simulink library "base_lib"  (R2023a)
settings: Solver=VariableStepAuto  StartTime=0.0  StopTime=10.0  RelTol=1e-3
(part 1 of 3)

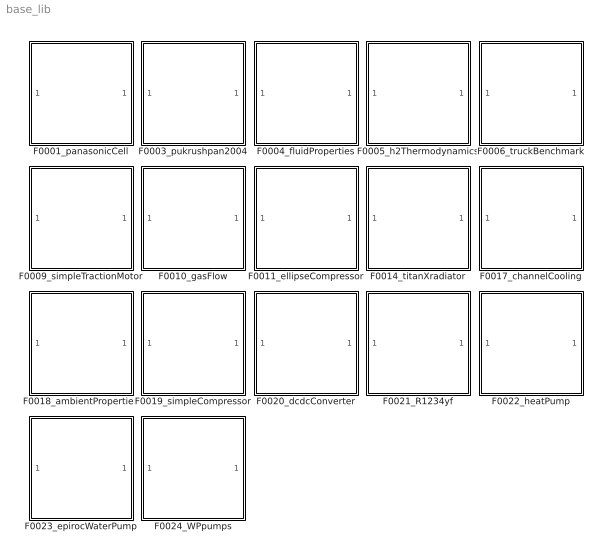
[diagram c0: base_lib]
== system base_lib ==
  F0001_panasonicCell : Subsystem
  F0003_pukrushpan2004 : Subsystem
  F0004_fluidProperties : Subsystem
  F0005_h2Thermodynamics : Subsystem
  F0006_truckBenchmark : Subsystem
  F0009_simpleTractionMotor : Subsystem
  F0010_gasFlow : Subsystem
  F0011_ellipseCompressor : Subsystem
  F0014_titanXradiator : Subsystem
  F0017_channelCooling : Subsystem
  F0018_ambientProperties : Subsystem
  F0019_simpleCompressor : Subsystem
  F0020_dcdcConverter : Subsystem
  F0021_R1234yf : Subsystem
  F0022_heatPump : Subsystem
  F0023_epirocWaterPump : Subsystem
  F0024_WPpumps : Subsystem

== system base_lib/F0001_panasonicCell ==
  F0001_cellCapacity.m : MATLAB Function  TreatAsAtomicUnit=on
  F0001_dynamicVoltage.m : MATLAB Function  TreatAsAtomicUnit=on
  F0001_ocvSOC.m : MATLAB Function  TreatAsAtomicUnit=on

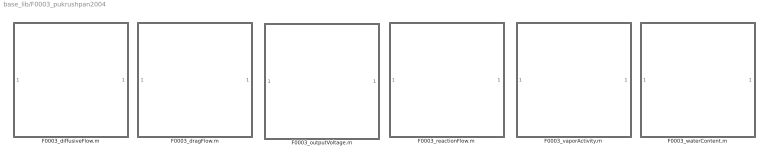
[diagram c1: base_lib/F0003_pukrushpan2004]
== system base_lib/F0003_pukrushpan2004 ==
  F0003_diffusiveFlow.m : MATLAB Function  TreatAsAtomicUnit=on
  F0003_dragFlow.m : MATLAB Function  TreatAsAtomicUnit=on
  F0003_outputVoltage.m : MATLAB Function  TreatAsAtomicUnit=on
  F0003_reactionFlow.m : MATLAB Function  TreatAsAtomicUnit=on
  F0003_vaporActivity.m : MATLAB Function  TreatAsAtomicUnit=on
  F0003_waterContent.m : MATLAB Function  TreatAsAtomicUnit=on

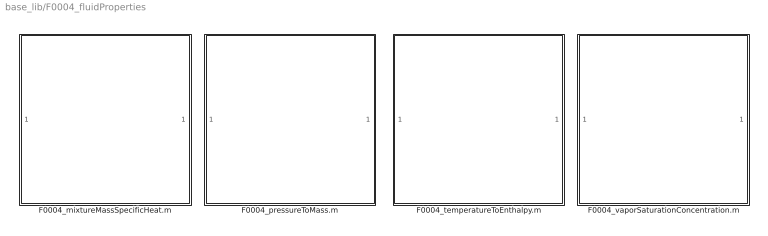
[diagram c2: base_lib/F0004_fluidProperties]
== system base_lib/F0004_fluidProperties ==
  F0004_mixtureMassSpecificHeat.m : MATLAB Function  TreatAsAtomicUnit=on
  F0004_pressureToMass.m : MATLAB Function  TreatAsAtomicUnit=on
  F0004_temperatureToEnthalpy.m : MATLAB Function  TreatAsAtomicUnit=on
  F0004_vaporSaturationConcentration.m : MATLAB Function  TreatAsAtomicUnit=on

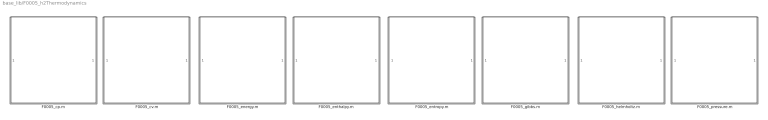
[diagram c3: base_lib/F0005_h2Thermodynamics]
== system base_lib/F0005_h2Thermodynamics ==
  F0005_cp.m : MATLAB Function  TreatAsAtomicUnit=on
  F0005_cv.m : MATLAB Function  TreatAsAtomicUnit=on
  F0005_energy.m : MATLAB Function  TreatAsAtomicUnit=on
  F0005_enthalpy.m : MATLAB Function  TreatAsAtomicUnit=on
  F0005_entropy.m : MATLAB Function  TreatAsAtomicUnit=on
  F0005_gibbs.m : MATLAB Function  TreatAsAtomicUnit=on
  F0005_helmholtz.m : MATLAB Function  TreatAsAtomicUnit=on
  F0005_pressure.m : MATLAB Function  TreatAsAtomicUnit=on

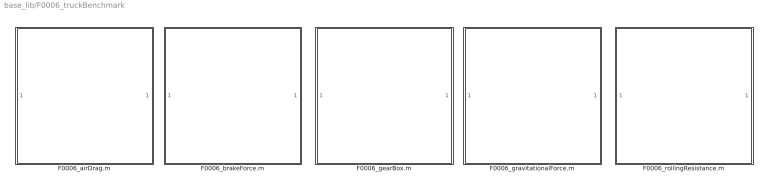
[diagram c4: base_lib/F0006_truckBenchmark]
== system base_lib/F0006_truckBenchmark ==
  F0006_airDrag.m : MATLAB Function  TreatAsAtomicUnit=on
  F0006_brakeForce.m : MATLAB Function  TreatAsAtomicUnit=on
  F0006_gearBox.m : MATLAB Function  TreatAsAtomicUnit=on
  F0006_gravitationalForce.m : MATLAB Function  TreatAsAtomicUnit=on
  F0006_rollingResistance.m : MATLAB Function  TreatAsAtomicUnit=on

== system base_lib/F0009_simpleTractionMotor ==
  F0009_currentDemand.m : MATLAB Function  TreatAsAtomicUnit=on
  F0009_torque.m : MATLAB Function  TreatAsAtomicUnit=on
  F0009_torqueLimit.m : MATLAB Function  TreatAsAtomicUnit=on

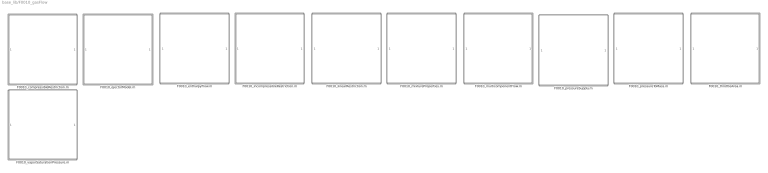
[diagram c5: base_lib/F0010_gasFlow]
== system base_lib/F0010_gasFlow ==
  F0010_compressibleRestriction.m : MATLAB Function  TreatAsAtomicUnit=on
  F0010_ejectorModel.m : MATLAB Function  TreatAsAtomicUnit=on
  F0010_enthalpyFlow.m : MATLAB Function  TreatAsAtomicUnit=on
  F0010_incompressibleRestriction.m : MATLAB Function  TreatAsAtomicUnit=on
  F0010_linearRestriction.m : MATLAB Function  TreatAsAtomicUnit=on
  F0010_mixtureProperties.m : MATLAB Function  TreatAsAtomicUnit=on
  F0010_multicomponentFlow.m : MATLAB Function  TreatAsAtomicUnit=on
  F0010_pressureSupply.m : MATLAB Function  TreatAsAtomicUnit=on
  F0010_pressureToMass.m : MATLAB Function  TreatAsAtomicUnit=on
  F0010_throttleArea.m : MATLAB Function  TreatAsAtomicUnit=on
  F0010_vaporSaturationPressure.m : MATLAB Function  TreatAsAtomicUnit=on

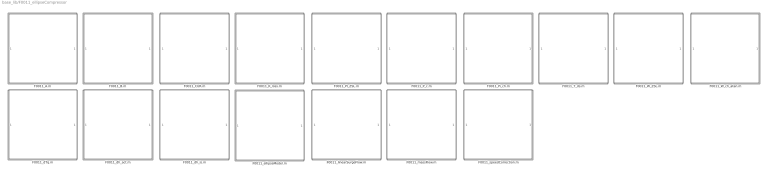
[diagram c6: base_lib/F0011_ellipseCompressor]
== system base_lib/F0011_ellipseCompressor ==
  F0011_A.m : MATLAB Function  TreatAsAtomicUnit=on
  F0011_B.m : MATLAB Function  TreatAsAtomicUnit=on
  F0011_CUR.m : MATLAB Function  TreatAsAtomicUnit=on
  F0011_K_loss.m : MATLAB Function  TreatAsAtomicUnit=on
  F0011_PI_ZSL.m : MATLAB Function  TreatAsAtomicUnit=on
  F0011_P_c.m : MATLAB Function  TreatAsAtomicUnit=on
  F0011_Pi_ch.m : MATLAB Function  TreatAsAtomicUnit=on
  F0011_T_ds.m : MATLAB Function  TreatAsAtomicUnit=on
  F0011_W_ZSL.m : MATLAB Function  TreatAsAtomicUnit=on
  F0011_W_ch_atan.m : MATLAB Function  TreatAsAtomicUnit=on
  F0011_dTq.m : MATLAB Function  TreatAsAtomicUnit=on
  F0011_dh_act.m : MATLAB Function  TreatAsAtomicUnit=on
  F0011_dh_is.m : MATLAB Function  TreatAsAtomicUnit=on
  F0011_ellipseModel.m : MATLAB Function  TreatAsAtomicUnit=on
  F0011_linearSurgeFlow.m : MATLAB Function  TreatAsAtomicUnit=on
  F0011_massFlow.m : MATLAB Function  TreatAsAtomicUnit=on
  F0011_speedCorrection.m : MATLAB Function  TreatAsAtomicUnit=on

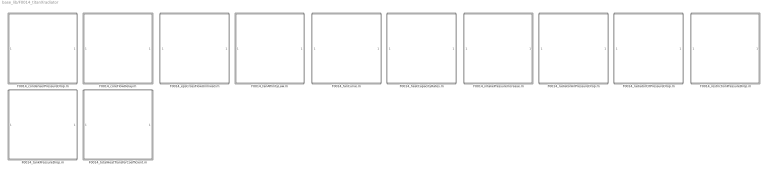
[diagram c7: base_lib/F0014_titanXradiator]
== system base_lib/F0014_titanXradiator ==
  F0014_condenserPressureDrop.m : MATLAB Function  TreatAsAtomicUnit=on
  F0014_coreFlowDelay.m : MATLAB Function  TreatAsAtomicUnit=on
  F0014_epsCrossFlowUnmixed.m : MATLAB Function  TreatAsAtomicUnit=on
  F0014_fanAffinityLaw.m : MATLAB Function  TreatAsAtomicUnit=on
  F0014_fanCurve.m : MATLAB Function  TreatAsAtomicUnit=on
  F0014_heatCapacityRates.m : MATLAB Function  TreatAsAtomicUnit=on
  F0014_intakePressureIncrease.m : MATLAB Function  TreatAsAtomicUnit=on
  F0014_radiatorAirPressureDrop.m : MATLAB Function  TreatAsAtomicUnit=on
  F0014_radiatorCltPressureDrop.m : MATLAB Function  TreatAsAtomicUnit=on
  F0014_restrictionPressureDrop.m : MATLAB Function  TreatAsAtomicUnit=on
  F0014_tankPressureDrop.m : MATLAB Function  TreatAsAtomicUnit=on
  F0014_totalHeatTransferCoefficient.m : MATLAB Function  TreatAsAtomicUnit=on

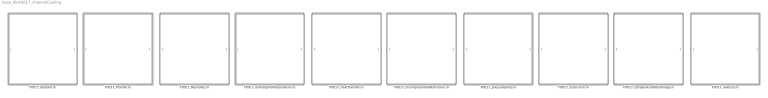
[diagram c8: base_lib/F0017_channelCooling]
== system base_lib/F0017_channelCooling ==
  F0017_Nusselt.m : MATLAB Function  TreatAsAtomicUnit=on
  F0017_Prandtl.m : MATLAB Function  TreatAsAtomicUnit=on
  F0017_Reynolds.m : MATLAB Function  TreatAsAtomicUnit=on
  F0017_enthalpyToTemperature.m : MATLAB Function  TreatAsAtomicUnit=on
  F0017_heatTransfer.m : MATLAB Function  TreatAsAtomicUnit=on
  F0017_incompressibleRestriction.m : MATLAB Function  TreatAsAtomicUnit=on
  F0017_pressureDrop.m : MATLAB Function  TreatAsAtomicUnit=on
  F0017_restriction.m : MATLAB Function  TreatAsAtomicUnit=on
  F0017_temperatureToEnthalpy.m : MATLAB Function  TreatAsAtomicUnit=on
  F0017_velocity.m : MATLAB Function  TreatAsAtomicUnit=on

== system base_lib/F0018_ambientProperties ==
  F0018_troposphereModel.m : MATLAB Function  TreatAsAtomicUnit=on

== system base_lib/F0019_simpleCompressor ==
  F0007_compressorPower.m : MATLAB Function  TreatAsAtomicUnit=on
  F0007_compressorTemperature.m : MATLAB Function  TreatAsAtomicUnit=on

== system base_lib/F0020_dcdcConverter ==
  F0020_dcdcConverter.m : MATLAB Function  TreatAsAtomicUnit=on

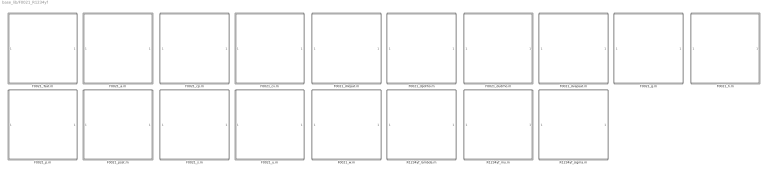
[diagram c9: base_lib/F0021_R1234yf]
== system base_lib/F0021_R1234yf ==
  F0021_Tsat.m : MATLAB Function  TreatAsAtomicUnit=on
  F0021_a.m : MATLAB Function  TreatAsAtomicUnit=on
  F0021_cp.m : MATLAB Function  TreatAsAtomicUnit=on
  F0021_cv.m : MATLAB Function  TreatAsAtomicUnit=on
  F0021_dliqsat.m : MATLAB Function  TreatAsAtomicUnit=on
  F0021_dpdrho.m : MATLAB Function  TreatAsAtomicUnit=on
  F0021_dudrho.m : MATLAB Function  TreatAsAtomicUnit=on
  F0021_dvapsat.m : MATLAB Function  TreatAsAtomicUnit=on
  F0021_g.m : MATLAB Function  TreatAsAtomicUnit=on
  F0021_h.m : MATLAB Function  TreatAsAtomicUnit=on
  F0021_p.m : MATLAB Function  TreatAsAtomicUnit=on
  F0021_psat.m : MATLAB Function  TreatAsAtomicUnit=on
  F0021_s.m : MATLAB Function  TreatAsAtomicUnit=on
  F0021_u.m : MATLAB Function  TreatAsAtomicUnit=on
  F0021_w.m : MATLAB Function  TreatAsAtomicUnit=on
  R1234yf_lambda.m : MATLAB Function  TreatAsAtomicUnit=on
  R1234yf_mu.m : MATLAB Function  TreatAsAtomicUnit=on
  R1234yf_sigma.m : MATLAB Function  TreatAsAtomicUnit=on

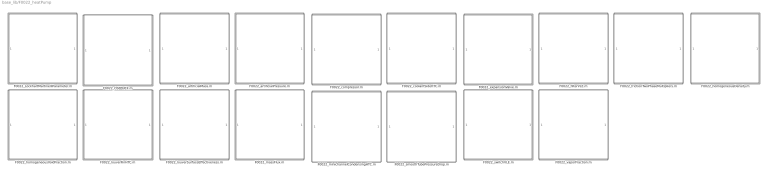
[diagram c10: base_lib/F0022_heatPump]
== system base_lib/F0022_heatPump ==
  F0022_LockhartMartinelliParameter.m : MATLAB Function  TreatAsAtomicUnit=on
  F0022_OSFPHEX.m : MATLAB Function  TreatAsAtomicUnit=on
  F0022_artificialMass.m : MATLAB Function  TreatAsAtomicUnit=on
  F0022_artificialPressure.m : MATLAB Function  TreatAsAtomicUnit=on
  F0022_compressor.m : MATLAB Function  TreatAsAtomicUnit=on
  F0022_coolantSideHTC.m : MATLAB Function  TreatAsAtomicUnit=on
  F0022_expansionValve.m : MATLAB Function  TreatAsAtomicUnit=on
  F0022_filterVLE.m : MATLAB Function  TreatAsAtomicUnit=on
  F0022_frictionTwoPhaseMultipliers.m : MATLAB Function  TreatAsAtomicUnit=on
  F0022_homogeneousDensity.m : MATLAB Function  TreatAsAtomicUnit=on
  F0022_homogeneousVoidFraction.m : MATLAB Function  TreatAsAtomicUnit=on
  F0022_louverFinHTC.m : MATLAB Function  TreatAsAtomicUnit=on
  F0022_louverSurfaceEffectiveness.m : MATLAB Function  TreatAsAtomicUnit=on
  F0022_massFlux.m : MATLAB Function  TreatAsAtomicUnit=on
  F0022_minichannelCondensingHTC.m : MATLAB Function  TreatAsAtomicUnit=on
  F0022_smoothTubePressureDrop.m : MATLAB Function  TreatAsAtomicUnit=on
  F0022_switchVLE.m : MATLAB Function  TreatAsAtomicUnit=on
  F0022_vaporFraction.m : MATLAB Function  TreatAsAtomicUnit=on

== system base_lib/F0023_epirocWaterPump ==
  F0023_current.m : MATLAB Function  TreatAsAtomicUnit=on
  F0023_pressure.m : MATLAB Function  TreatAsAtomicUnit=on
  F0023_speed.m : MATLAB Function  TreatAsAtomicUnit=on

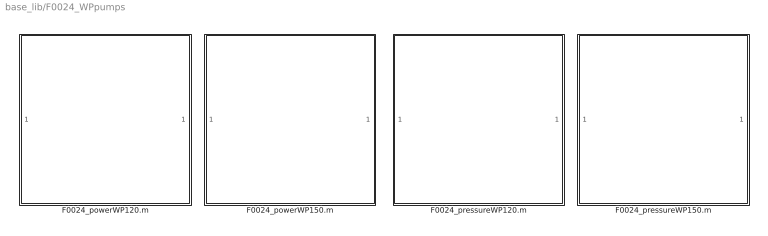
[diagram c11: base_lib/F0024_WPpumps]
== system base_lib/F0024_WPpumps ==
  F0024_powerWP120.m : MATLAB Function  TreatAsAtomicUnit=on
  F0024_powerWP150.m : MATLAB Function  TreatAsAtomicUnit=on
  F0024_pressureWP120.m : MATLAB Function  TreatAsAtomicUnit=on
  F0024_pressureWP150.m : MATLAB Function  TreatAsAtomicUnit=on

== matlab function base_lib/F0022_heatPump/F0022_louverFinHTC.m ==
function h = F0022_louverFinHTC(u, par)

% HEX Geometry
% L_a = 23;       % Louver angle [degrees]
% F_p = 1.4e-3;   % Fin pitch [m]
% L_p = 1.7e-3;   % Louver pitch [m]
% L_l = 6.4e-3;   % Louver length [m]
% H   = 8.15e-3;  % Fin height [m]
% T_p = 10.15e-3; % Tube pitch [m]
% T_d = 16e-3;    % Tube depth [m]
% d_f = 0.1e-3;   % Fin thickness [m]
% F_d = 16e-3;    % flow depth

% contraction ratio
sigma = par.sigma;

% Air properties
cp  = par.cp_air;
v   = par.v_air;
rho = par.rho_air;

% HEX Geometry parameters
L_a  = par.L_a;  % Louver angle [deg]
F_p  = par.F_p;  % Fin pitch [m]
L_p  = par.L_p;  % Louver pitch [m]
L_l  = par.L_l;  % Louver length [m]
H    = par.H;    % Fin height [m]
T_p  = par.T_p;  % Tube pitch [m]
% T_d  = par.T_d;  % Tube depth [m]
d_f  = par.d_f;  % Fin thickness [m]
F_d  = par.F_d;  % Flow depth [m]

% Prandtl number
P_r = 0.7;

% minimum air velocity
u = max(0.001, u);

% maximum air velocity
V_c = u .* sigma;

% Air side Reynolds number based on Louver pitch
Re = V_c .* L_p ./ v;

% Colburn j-factor correlation
j = Re.^(-0.487) .* (L_a./90).^(0.257) * ...
    (F_p./L_p).^(-0.13) .* (H ./ L_p).^(-0.29) .* ...
    (F_d ./ L_p).^(-0.235) .* (L_l./L_p).^(0.68) .* ...
    (T_p./L_p).^(-0.279) .* (d_f./L_p).^(-0.05);


% HTC
h = j .* rho .* V_c .* cp ./ P_r.^(2/3);

end

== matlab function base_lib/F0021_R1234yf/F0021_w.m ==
function w = F0021_w(T,rho)
%R1234yf_w
%    W = R1234yf_w(T,RHO)

%    This function was generated by the Symbolic Math Toolbox version 9.3.
%    16-Oct-2023 15:47:53

t2 = T.^2;
t3 = rho.^2;
t4 = rho.^3;
t6 = rho.^5;
t8 = rho.^7;
t9 = 1.0./T;
t12 = rho./4.17e+3;
t17 = rho.*7.769784172661871e-3;
t25 = rho.*4.892086330935252e-4;
t30 = rho.*2.800959232613909e-3;
t32 = rho.*6.407673860911271e-4;
t33 = rho.*5.059952038369305e-4;
t5 = t3.^2;
t7 = t3.^3;
t10 = 1.0./t2;
t11 = t9.^3;
t13 = t9.*7.18e+2;
t14 = t9.*8.77e+2;
t15 = t9.*1.755e+3;
t16 = t9.*4.465e+3;
t18 = -t12;
t23 = t9.*5.8856e+4;
t31 = t9.*3.6785e+2;
t34 = t9.*7.94556e+4;
t35 = t3./1.73889e+7;
t40 = t9.*1.044694e+3;
t41 = t12-4.1e+1./2.5e+1;
t49 = t9.*6.54773e+2;
t50 = t9.*1.699467e+3;
t51 = t12-9.1e+1./1.0e+2;
t52 = t12-8.9e+1./1.25e+2;
t53 = t12-3.59e+2./5.0e+2;
t68 = t12-6.77e+2./1.0e+3;
t69 = t17-5.3136e+1;
t78 = t25-1.45248;
t87 = t30-8.38624;
t92 = t32-2.43152;
t100 = t33-1.42847;
t123 = t4.*t9.*9.319180196722149e-10;
t19 = -t13;
t20 = -t14;
t21 = -t15;
t22 = -t16;
t24 = exp(t18);
t42 = -t35;
t43 = t31.^(3.0./2.0);
t44 = t31.^(2.0./5.0);
t45 = t31.^(5.0./2.0);
t46 = t31.^(7.0./2.0);
t47 = t31.^(7.0./5.0);
t54 = t31-6.0./5.0;
t55 = t31.^(1.0./2.0e+1);
t56 = t41.^2;
t57 = t31.^(8.0./2.5e+1);
t59 = t31.^(1.9e+1./2.5e+1);
t61 = t31.^(3.6e+1./2.5e+1);
t62 = t31.^(1.9e+1./5.0e+1);
t63 = t31.^(4.4e+1./2.5e+1);
t65 = t31.^(6.1e+1./2.5e+1);
t66 = t31.^(4.7e+1./5.0e+1);
t67 = t23-2.048e+2;
t70 = t31-3.2e+1./2.5e+1;
t71 = t31-2.3e+1./5.0e+1;
t72 = 1.0./t31.^(3.0./1.0e+2);
t73 = t51.^2;
t74 = t52.^2;
t75 = t53.^2;
t77 = t31.^(9.7e+1./1.0e+2);
t79 = t31-6.7e+1./1.0e+2;
t80 = t31-1.13e+2./1.0e+2;
t81 = t34-2.592e+2;
t82 = t68.^2;
t85 = t31.^(9.29e+2./1.0e+3);
t97 = t40-3.2092;
t103 = t49-8.188e-1;
t106 = t50-3.0954;
t26 = exp(t19);
t27 = exp(t20);
t28 = exp(t21);
t29 = exp(t22);
t48 = exp(t42);
t58 = t55.^21;
t60 = t57.^4;
t64 = t59.^3;
t76 = t54.^2;
t83 = t70.^2;
t84 = t71.^2;
t88 = t79.^2;
t89 = t80.^2;
t90 = t56.*(8.1e+1./5.0);
t95 = t74.*(5.1e+1./5.0e+1);
t99 = t75.*(1.46e+2./2.5e+1);
t101 = t73.*(1.67e+2./1.25e+2);
t107 = t82.*(2.11e+2./2.0e+2);
t115 = t57.*1.546958;
t119 = t85.*2.355237;
t120 = rho.*t66.*2.315508393285372e-4;
t130 = t3.*t62.*3.033007263254145e-8;
t133 = rho.*t24.*t77.*3.263914628297362e-4;
t136 = t3.*t24.*t77.*3.913566700596357e-8;
t36 = t26-1.0;
t37 = t27-1.0;
t38 = t28-1.0;
t39 = t29-1.0;
t86 = t76.*1.08e+2;
t93 = -t90;
t94 = t83.*8.0e+1;
t98 = -t95;
t102 = -t99;
t104 = -t101;
t105 = t84.*(8.9e+1./1.0e+2);
t109 = t89.*(7.1e+1./5.0e+1);
t110 = -t107;
t112 = t88.*(2.31e+2./1.0e+2);
t121 = -t119;
t122 = -t120;
t131 = t48.*t64.*1.210006;
t134 = rho.*t48.*t65.*3.342232613908873e-4;
t137 = t3.*t48.*t64.*1.391699302428561e-7;
t138 = -t136;
t139 = t3.*t48.*t63.*1.06569432224005e-7;
t141 = t4.*t48.*t65.*1.922049476337705e-11;
t142 = t5.*t48.*t63.*4.085726420264459e-15;
t143 = t7.*t24.*t58.*3.588938332192827e-23;
t145 = t8.*t24.*t58.*1.229509534838242e-27;
t91 = -t86;
t96 = -t94;
t108 = -t105;
t111 = -t109;
t113 = -t112;
t132 = -t131;
t135 = -t134;
t140 = -t139;
t144 = -t143;
t114 = t91+t93;
t117 = t96+t102;
t124 = t98+t111;
t126 = t104+t113;
t127 = t108+t110;
t116 = exp(t114);
t118 = exp(t117);
t125 = exp(t124);
t128 = exp(t126);
t129 = exp(t127);
t146 = t3.*t9.*t118.*7.283294189396684e-5;
t148 = rho.*t46.*t116.*1.644384172661871e-7;
t149 = t47.*t125.*1.389966;
t150 = t11.*t128.*2.377824987227386e+7;
t152 = t3.*t46.*t129.*3.407663509480186e-8;
t154 = t4.*t9.*t87.*t118.*5.821977769301905e-9;
t155 = t3.*t46.*t69.*t116.*1.971683660266032e-11;
t157 = rho.*t47.*t78.*t125.*3.333251798561151e-4;
t159 = rho.*t11.*t92.*t128.*5.702218194789895e+3;
t160 = t4.*t46.*t100.*t129.*2.723951646267135e-12;
t147 = -t146;
t151 = -t150;
t153 = -t152;
t156 = -t155;
t158 = -t157;
t161 = t115+t121+t122+t123+t130+t132+t133+t135+t137+t138+t140+t141+t142+t144+t145+t147+t148+t149+t151+t153+t154+t156+t158+t159+t160;
et1 = t66.*9.65567e-1+t138+t145-rho.*t62.*2.529528057553957e-4-t3.*t9.*1.165829442609941e-5-t24.*t77.*1.3610524;
et2 = t48.*t65.*1.393711-t46.*t116.*6.857082e-4+t87.*t154+t92.*t159+t100.*t160+rho.*t24.*t77.*6.527829256594724e-4+rho.*t48.*t63.*8.887890647482015e-4;
et3 = rho.*t48.*t64.*(-1.741015827338129e-3)+rho.*t9.*t118.*6.074267353956834e-1-rho.*t11.*t128.*1.52363270164786e+4+rho.*t47.*t125.*6.799833669064748e-4;
et4 = rho.*t46.*t129.*2.841991366906475e-4+t6.*t24.*t58.*8.979523707146454e-19-t7.*t24.*t58.*7.177876664385654e-23;
et5 = t4.*t48.*t63.*(-1.192623542075196e-10)-t3.*t48.*t65.*4.007473158164116e-7+t4.*t48.*t64.*6.674816798218516e-11+t6.*t48.*t63.*1.95958101691341e-18;
et6 = t5.*t48.*t65.*9.218462716247988e-15-t4.*t9.*t118.*6.800070034544626e-8+t3.*t46.*t116.*6.388255059261943e-10;
et7 = t4.*t46.*t129.*(-5.747537973623655e-12)-t11.*t92.*t128.*4.755649974454772e+7+t47.*t78.*t125.*2.779932+rho.*t46.*t69.*t116.*3.288768345323741e-7;
et8 = t3.*t9.*t87.*t118.*(-1.456658837879337e-4)-t3.*t46.*t100.*t129.*6.815327018960372e-8-rho.*t47.*t78.^2.*t125.*3.333251798561151e-4-t3.*t46.*t69.^2.*t116.*1.971683660266032e-11;
et9 = t4.*2.533418566459739e-12-t48.*t60.*2.75881368-t3.*t118.*1.979963079895795e-7-t10.*t128.*1.93923473200548e+5;
et10 = t44.*t125.*1.9459524+t67.*t146+t81.*t155+t97.*t157+t103.*t152+t106.*t150-rho.*t72.^2.*2.176577889688249e-4+t3.*1.0./t31.^(3.1e+1./5.0e+1).*1.152542760036575e-8+1.0./t31.^(1.7e+1./2.5e+1).*4.9502656e-1;
et11 = 1.0./t31.^(7.1e+1./1.0e+3).*(-2.188015173)+rho.*t24.*t72.*3.165997189448441e-4-rho.*t48.*t61.*8.155047577937649e-4+rho.*t45.*t116.*5.755344604316547e-7;
et12 = t7.*t24.*t55.*(-3.768385248802469e-23)+t8.*t24.*t55.*1.290985011580154e-27-t3.*t24.*t72.*3.796159699578467e-8;
et13 = t3.*t48.*t59.*(-1.875622007142488e-7)+t3.*t48.*t60.*3.173074409537118e-7+t5.*t48.*t59.*7.190878499665448e-15+t4.*t48.*t61.*4.689800722264001e-11;
et14 = t3.*t45.*t129.*(-1.192682228318065e-7)+t4.*t87.*t118.*1.582704300476255e-11-t47.*t97.*t125.*1.389966+rho.*t10.*t92.*t128.*4.650443002411223e+1;
et15 = rho.*t46.*t81.*t116.*(-1.644384172661871e-7)-rho.*t44.*t78.*t125.*4.666552517985612e-4-t3.*t45.*t69.*t116.*6.900892810931111e-11+t4.*t45.*t100.*t129.*9.533830761934972e-12;
et16 = rho.*t11.*t92.*t106.*t128.*(-5.702218194789895e+3)-t4.*t9.*t67.*t87.*t118.*5.821977769301905e-9-t4.*t46.*t100.*t103.*t129.*2.723951646267135e-12;
et17 = t2.*3.653734124219459e-5+1.0./t36.^2.*exp(t9.*-1.436e+3).*2.876052391546904e+1+1.0./t37.^2.*exp(t9.*-1.754e+3).*8.736380352244283+1.0./t38.^2.*exp(t9.*-3.51e+3).*1.696916093943165e+2+1.0./t39.^2.*exp(t9.*-8.93e+3).*2.990869359808914e+2+rho.*t72.^56.*8.072375558752998e-5;
et18 = rho.*1.0./t31.^1.071.*(-3.72539753676259e-5)-(t26.*2.876052391546904e+1)./t36-(t27.*8.736380352244283)./t37-(t28.*1.696916093943165e+2)./t38-(t29.*2.990869359808914e+2)./t39;
et19 = t4.*t72.^54.*5.712042455816759e-13-t3.*1.0./t31.^(5.3e+1./5.0e+1).*1.565883373876438e-9+rho.*t31.^(7.0./2.5e+1).*t48.*8.468300984172661e-4;
et20 = rho.*1.0./t55.^12.*t125.*(-1.866621007194245e-4)+t8.*t24.*1.0./t55.^19.*6.454925057900768e-29+t3.*t31.^(1.1e+1./2.5e+1).*t48.*1.408065768852544e-7;
et21 = t4.*t48.*t72.^8.*1.139466607056987e-11+t3.*t24.*1.0./t31.^(1.03e+2./1.0e+2).*1.13884790987354e-9+rho.*t9.*t128.*2.528445291510791e-1;
et22 = rho.*t11.*t128.*(-2.634424805992931e+4)+rho.*t47.*t125.*9.466435107913669e-4-t4.*t9.*t118.*9.315164430883049e-7;
et23 = t3.*t43.*t116.*(-1.725223202732778e-10)+t3.*t46.*t116.*4.258836706174629e-9+t4.*t43.*t129.*2.383457690483743e-11-t4.*t46.*t129.*4.8486339303555e-12;
et24 = t4.*t67.*t118.*(-3.165408600952511e-11)-rho.*t10.*t106.*t128.*9.300886004822446e+1+rho.*t44.*t97.*t125.*9.333105035971223e-4+t3.*t45.*t81.*t116.*1.380178562186222e-10;
et25 = t4.*t45.*t103.*t129.*(-1.906766152386994e-11)+rho.*t11.*t106.^2.*t128.*5.702218194789895e+3-rho.*t47.*t97.^2.*t125.*3.333251798561151e-4;
et26 = t4.*t9.*t67.^2.*t118.*5.821977769301905e-9-t3.*t46.*t81.^2.*t116.*1.971683660266032e-11+t4.*t46.*t103.^2.*t129.*2.723951646267135e-12;
w = sqrt(T.*((rho.*t161)./2.085e+3-(t3.*(et1+et2+et3+et4+et5+et6+et7+et8))./1.73889e+7+(t2.*(t12.*t161-rho.*t9.*(et9+et10+et11+et12+et13+et14+et15+et16).*8.821342925659472e-2+1.0).^2.*7.39023892439211e-6)./(et17+et18+et19+et20+et21+et22+et23+et24+et25+et26)+1.0).*7.290736472421491e+1);
end

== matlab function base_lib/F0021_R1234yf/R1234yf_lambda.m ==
function lambda = R1234yf_lambda(T, rho, cp, cv, mu, dp_drho, dp_drho_R)


% Critical point & molar mass
Tc   =     367.85; % [K]
pc   = 	3382200.0; % [Pa]
rhoc =     4170.0; % [mol/m3]
M    = 0.1140415928; % [kg/mol]
% R    = 8.314472;

% change units
rhoc = rhoc .* M;
rho  = rho  .* M;

% coefficients
A = [-0.0102778; 0.0291098; 0.000860643];

B      = zeros(5,2);
B(1,1) = -0.0368219;
B(1,2) =  0.0397166;
B(2,1) =  0.0883226;
B(2,2) = -0.0772390;
B(3,1) = -0.0705909;
B(3,2) =  0.0664707;
B(4,1) =  0.0259026;
B(4,2) = -0.0249071;
B(5,1) = -0.00322950;
B(5,2) =  0.00336228;


% Dilute-gas thermal conductivity
lambda_0 = sum( repmat(A', length(T), 1) .* (T./Tc).^(0:2), 2 );

% residual thermal conductivity
lambda_r = sum( (  repmat(B(:,1)', length(T), 1) + ...
    repmat(B(:,2)', length(T), 1) .* repmat((T./Tc), 1, 5) ) .* ...
    (rho./rhoc).^(1:5), 2);

% critical enhancement
R0        = 1.03;
kb        = 1.380649e-23;
eta       = mu;
T_R       = 1.5 .* Tc;
gam       = 1.239;
nu        = 0.63;
GAM       = 0.0496;
xi0       = 1.94e-10;
qd        = 0.5835e9;
dp_drho   = dp_drho   ./ M;
dp_drho_R = dp_drho_R ./ M;
drho_dp   = 1 ./ dp_drho;
drho_dp_R = 1 ./ dp_drho_R;


xi = xi0 .* ( pc .* rho ./ (GAM .* rhoc.^2) ).^(nu./gam) .* ...
            (  drho_dp - (T_R./T) .* drho_dp_R  ).^(nu./gam);


omega0    = 2./pi .* (1 - exp(-1./ ( 1./(qd.*xi) + (1/3) .* (qd.*xi.*rhoc./rho).^2 ) ) );
omega     = 2./pi .* (  (cp-cv)./cp .* atan(qd.*xi) + cv./cp .* qd.*xi );
dlambda_c = rho .* cp .* R0 .* kb .* T ./ (6 .* pi .* eta .* xi) .* (omega-omega0);

lambda = lambda_0 + lambda_r + dlambda_c;

end

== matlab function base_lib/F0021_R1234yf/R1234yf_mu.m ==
function mu = R1234yf_mu(T,rho)

% Critical point & molar mass
Tc   =     367.85; % [K]
% pc   = 	3382200.0; % [Pa]
rhoc =     4170.0; % [mol/m3]
% M    = 0.1140415928; % [kg/mol]
% R    = 8.314472;

% Viscosity coefficients
a0 = -836950;
a1 = 6336.28;
a2 = -2.3547;
a3 = 0.0395563;
a4 = 39509.1;
a5 = 121.018;

b0 = -19.572881;
b1 = 219.73999;
b2 = -1015.3226;
b3 = 2471.0125;
b4 = -3375.1717;
b5 = 2491.6597;
b6 = -787.26086;
b7 = 14.085455;
b8 = -0.34664158;

b = [b0; b1; b2; b3; b4; b5; b6];

c0 = -0.19425910;
c1 = -2.079577245;
c2 = 0;
c3 = -43.47027288;
c4 = 0;
c5 = 0;
c6 = 0;
c7 = -3.53682791;
c8 = 1;

% dilute-gas limit viscosity
eta0 = (a0 + a1 .* T + a2 .* T.^2 + a3 .* T.^3) ./ (a4 + a5 .* T + T.^2);

% temperature dependent contribution
sigma   = 0.531e-9;
e_kb    = 275;
Mw      = 114.0416e-3;
N_a     = 6.02214076e23;
T_star  =  T ./ e_kb;
Bn_star = sum(  repmat(b', length(T), 1) .* T_star.^(-0.25.*(0:6)) , 2) + b7 .* T_star.^(-2.5) + b8 .* T_star.^-5.5; 
Bn      = Bn_star .* N_a .* sigma.^3;
eta1    = Bn .* eta0;

% residual term
rhor = rho ./ rhoc;
Tr    = T ./ Tc;

deta = rhor.^(2/3) .* Tr.^(1/2) .* ...
                (c0 + c1 .* rhor + c2 .* rhor.^2 +  ... 
                        (c3 .* rhor + c4 .* rhor.^6 + c5 .* rhor .* Tr.^2 + c6 .* rhor.^5 .* Tr) ./ (c7 .* Tr + c8 .* rhor .* Tr) );


% total viscosity
eta = eta0 + eta1 .* rho + deta;

% SI units
mu = eta .* 1e-6;

end

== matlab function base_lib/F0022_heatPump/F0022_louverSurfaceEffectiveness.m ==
function eta = F0022_louverSurfaceEffectiveness(h, par)

% HEX Geometry parameters
H    = par.H;    % Fin height [m]
d_f  = par.d_f;  % Fin thickness [m]
F_d  = par.F_d;  % Flow depth [m]

% Areas
A_f = par.A_f;
A_o = par.A_o;


% aluminium properties
k = par.k_w;


% Fin efficiency
m     = sqrt( 2.*h ./ (k .* d_f) .* (1 + d_f./F_d) );
l     = H/2 - d_f;
eta_f = tanh(m*l) ./ m.*l;

% Surface effectiveness
eta   = 1 - A_f ./ A_o .* (1 - eta_f);

end

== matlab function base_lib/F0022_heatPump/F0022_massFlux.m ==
function G = F0022_massFlux(W, par)

% parameters
D_h = par.D_h;

% mass flux
G = 4 .* W ./ (D_h.^2 .* pi);
end

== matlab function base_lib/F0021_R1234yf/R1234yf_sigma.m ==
function sigma = R1234yf_sigma(T)

% Critical point & molar mass
Tc   =     367.85; % [K]
% pc   = 	3382200.0; % [Pa]
% rhoc =     4170.0; % [mol/m3]
% M    = 0.1140415928; % [kg/mol]
% R    = 8.314472;

% max & min temperature
T = max(T,  0);
T = min(T, Tc);

% coefficients
c = [ 42.36234 0.60895 -0.42621 367.85]';

% surface tension
Tr      = T ./ Tc; 
sigma = c(1) .* (1 - Tr).^1.26 .* ( 1 + c(2).*(1-Tr).^0.5 + c(3).*(1-Tr) );

% shift to SI unit
sigma = sigma * 1e-3;

end

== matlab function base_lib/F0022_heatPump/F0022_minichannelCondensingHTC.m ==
function h = F0022_minichannelCondensingHTC(G, p_sat,  x, rho_f, rho_g, cp_f, cp_g, mu_f, mu_g, k_f, k_g, par)
% Critical point & molar mass
pc = par.pc;

% gravity
g = 9.82;

% channel dimensions
b = par.b;
a = par.a;

% hydraulic diameter
D_h =  2 .* a .* b ./ (a + b);

G = max(G,0);

% Liquid reynolds & prandtl numbers
Re_f = (1-x) .* G .* D_h ./ mu_f;
Pr_f = cp_f .* mu_f ./ k_f;

% liquid only heat transfer coefficient
h_f = 0.023 .* Re_f.^0.8 .* Pr_f.^0.4 .* k_f ./ D_h;

% Gas only reynolds & prandtl numbers
Re_g = x .* G .* D_h ./ mu_g;
Pr_g = cp_g .* mu_g ./ k_g;



% gas only heat transfer coefficient
h_g = 0.023 .* Re_g.^0.8 .* Pr_g.^0.4 .* k_g ./ D_h;

% reduced pressure
p_r = p_sat ./ pc;

% Shah correlating parameter
% Z = (1./max(min(x,1),0.0000001) - 1).^0.8 .* p_r.^0.4;

Z = ( (1-x)./(x+0.00001) ).^0.8 .* p_r.^0.4;

% Regime depenedent HTCs
h_I = h_f .* (1 + 3.8./(Z.^0.95 + 0.00001)) .* ...
    (mu_f ./ (14 .* mu_g)).^(0.0058 + 0.557 .* p_r);


% smooth transition to subcooled liquid & superheated vapor
y = (x-0.1) / 0.1;
y = tanh(y*5)/2 + 1/2;
z =  (x-0.90) / 0.1;
z = tanh(z*5)/2 + 1/2;

% HTC
h = h_I .* y .* (1-z) + h_f .* (1-y) + h_g .* z;


% h_nu = 1.32 .* Re_f.^(-1/3) .* ...
%     (  rho_f .* (rho_f - rho_g) .* g .* k_f.^3 ./ mu_f.^2   ).^(1/3);
% 
% % dimensionless vapor velocity
% J_g = x.*G ./ (g.*D_h.*rho_g.*(rho_f - rho_g)).^0.5;
% 
% % Single phase regimes
% SP_REG1 = x == 0;
% SP_REG2 = x == 1;
% TP_REG1 = (~SP_REG1) & (~SP_REG2);
% 
% % % Two-phase regimes
% % TP      =  (x>0) & (x<1); 
% 
% % % vertical flow
% % TP_REG1 = TP & (J_g >= 1./(2.4.*Z + 0.73));
% % TP_REG3 = TP & (J_g <= 0.89 - 0.93 .* exp(-0.987 .* Z.^(-1.17)));
% % TP_REG2 = TP & (~TP_REG1 & ~TP_REG3);
% 
% % % horizontal flow
% % TP_REG1 = TP & (J_g >= 0.98 .* (Z + 0.263).^(-0.62) );
% % TP_REG3 = TP & (J_g <= 0.95 .* (1.254 + 2.27 .* Z.^1.249 ).^(-1) );
% % TP_REG2 = TP & (~TP_REG1 & ~TP_REG3);
% 
% % Output
% h = zeros(size(x));
% h( SP_REG1 ) = h_f( SP_REG1 );
% h( SP_REG2 ) = h_g( SP_REG2 );
% h( TP_REG1 ) = h_I( TP_REG1 );
% % h( TP_REG2 ) = h_I( TP_REG2 ) + h_nu( TP_REG2 );
% % h( TP_REG3 ) = h_nu( TP_REG3 );

end

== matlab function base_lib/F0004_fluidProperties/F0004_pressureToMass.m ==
function m = F0004_pressureToMass(p, T, par)
% gas constants
R_r    = par.R_r;
R_H2O  = par.R_H2O;
R_N2   = par.R_N2;
Rj     = [R_r; R_H2O; R_N2];
V      = par.V;

% mass
m = p .* V ./ (Rj .* T);
end

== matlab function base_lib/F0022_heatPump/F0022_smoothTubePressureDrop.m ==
function dp = F0022_smoothTubePressureDrop(W, x, rho_f, rho_g, mu_f, mu_g, sigma, par)

% parameters
D = par.D;
L = par.L;

% gravitation
g = 9.82;

% minimum mass flux
W = max(W, 1e-4);

% mass flux
G_tp = 4.*W ./ (pi.*D.^2);

% liquid-only friction factor
Re_lo = G_tp .* D ./ mu_f;
f_lo  = 0.25 .* ( log10(  150.39 ./ (Re_lo.^0.98865) - 152.66./(Re_lo)  ) ).^(-2);

% gas-only friction factor
Re_go = G_tp .* D ./ mu_g;
f_go  = 0.25 .* ( log10(  150.39 ./ (Re_go.^0.98865) - 152.66./(Re_go)  ) ).^(-2);

% Laplace constant
La = sqrt( sigma ./ (g.*(rho_f - rho_g) ) ) ./ D;

% liquid-only pressure gradient
dp_dz_lo = G_tp.^2 ./(2.*D.*rho_f) .* f_lo;

% gas-only pressure gradient
dp_dz_go = G_tp.^2 ./(2.*D.*rho_g) .* f_go;

% two phase multiplier
Y       = sqrt(dp_dz_go ./ dp_dz_lo);
phi2_lo = (Y.^2 .* x.^3 + (1-x).^(1/3) .* (1+2.*x.*(Y.^2 -1)) ) .* ...
    (1 + 1.54 .*(1-x).^0.5 .* La.^1.47); 

% two-phase pressure gradient
dp_dz_tp = dp_dz_lo .* phi2_lo; 

% pressure drop
dp = dp_dz_tp .* L;

end

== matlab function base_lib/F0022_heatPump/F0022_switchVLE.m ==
function y = F0022_switchVLE(x)
% step function on 0-1
y = tanh( 1000*(x-0.01) ) / 2  - tanh( 1000*(x-0.99) ) / 2;

end

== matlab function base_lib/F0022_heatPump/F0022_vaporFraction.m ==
function x = F0022_vaporFraction(B, B_liq, B_vap)

% B is an arbitrary thermodynamic property, ie
% specific volume, enthalpy, etc.

x = (B - B_liq) ./ (B_vap - B_liq);

end

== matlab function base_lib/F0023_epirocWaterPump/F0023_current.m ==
function I = F0023_current(q, V)

% parameters
a = [-4.6456; 2.8036; 1.7966];

% function
I = a(1) + a(2) .* q + a(3) .* V; 

end

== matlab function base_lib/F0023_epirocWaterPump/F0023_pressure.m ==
function dp = F0023_pressure(q, V)

% parameters
a = [-0.1990; 0.2290; 0.1984; -0.0313; -0.2935];

% function
dp = a(1) + a(2) .* q + a(3) .* V + a(4) .* q.* V + a(5) .* q.^2;

end

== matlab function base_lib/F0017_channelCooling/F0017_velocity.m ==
function v = F0017_velocity(W, par)

% parameters
rho = par.rho_clt;
d   = par.d;

% area
A = pi .* d.^2 / 4;

% velocity
v = W ./ (rho .* A);

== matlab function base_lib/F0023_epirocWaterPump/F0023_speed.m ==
function w = F0023_speed(q, V)

% parameters
b = [1.6954; 0.3962; 0.4124; -0.0700];

% function
w = 1000 * (b(1) + b(2) .* q + b(3) .* V + b(4) .* q.* V) .* 2.*pi/60; 

end

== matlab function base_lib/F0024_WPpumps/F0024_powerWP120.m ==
function P = F0024_powerWP120(q, n)

% parameters
a = [-385.2919; 155.7472; 0.1219];

% function
P = a(1) + a(2) .* q + a(3) .* n; 

end

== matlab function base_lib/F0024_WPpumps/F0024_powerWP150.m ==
function P = F0024_powerWP150(q, n)

% parameters
a =  [-1578.62293476575; 122.984201937838; 0.569192422324180];

% function
P = a(1) + a(2) .* q + a(3) .* n; 

end

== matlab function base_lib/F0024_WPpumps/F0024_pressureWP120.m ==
function dp = F0024_pressureWP120(q, n)

% parameters
a = 1.0e+04 * [0.8098; 0.0038; 0.0013; -5.4000];

% function
dp = a(1) + a(2) .* n + a(3) .* q.* n + a(4) .* q.^2;

end

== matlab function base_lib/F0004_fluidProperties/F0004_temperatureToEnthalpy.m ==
function h = F0004_temperatureToEnthalpy(T, par)
% output size
h = zeros(3,1);

% mass heat capacity
cp_r  = par.cp_r;
cp_v  = par.cp_H2O;
cp_N2 = par.cp_N2;
cp    = [cp_r; cp_v; cp_N2];

% specific enthalpy
h = cp .* T;
end

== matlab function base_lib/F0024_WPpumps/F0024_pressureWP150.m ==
function dp = F0024_pressureWP150(q, n)

% parameters
a = [-123461.665683305;
    69.1858073291126; 3.37203190426057; -3645.86929609208];

% function
dp = a(1) + a(2) .* n + a(3) .* q.* n + a(4) .* q.^2;

end

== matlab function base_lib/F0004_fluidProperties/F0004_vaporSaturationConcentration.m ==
function c_sat = F0004_vaporSaturationConcentration(p_sat, T, par)
% saturation concentration
c_sat = p_sat ./ (par.R .* T);

end

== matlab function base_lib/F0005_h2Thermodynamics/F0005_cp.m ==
function cp = F0005_cp(T,rho)
%ISOBARICHEATCAPACITY
%    CP = ISOBARICHEATCAPACITY(T,RHO)

%    This function was generated by the Symbolic Math Toolbox version 8.7.
%    04-Nov-2021 19:06:05

t2 = rho.^2;
t3 = rho.^3;
t4 = 1.0./T;
t5 = rho./1.5508e+4;
t9 = rho.*2.17307196285788e-4;
t10 = rho.*1.328346659788496e-5;
t11 = rho.*6.30642249161723e-5;
t12 = rho.*3.231880319834924e-4;
t13 = rho.*2.072478720660304e-4;
t6 = -t5;
t8 = t4.*3.3145e+1;
t14 = t5-3.9e+1./2.5e+2;
t15 = t5-6.7e+1./1.0e+2;
t16 = t5-2.17e+2./1.25e+2;
t17 = t4.*8.644216;
t18 = t4.*1.133559e+1;
t19 = t4.*1.4882105e+1;
t20 = t4.*1.8461765e+1;
t21 = t5-7.53e+2./5.0e+2;
t22 = t5-8.31e+2./5.0e+2;
t26 = t4.*2.6297243e+1;
t53 = t10-3.57616e-1;
t59 = t9-5.07522;
t60 = t11-1.52568e-1;
t61 = t12-3.35804;
t68 = t13-5.341668;
t69 = t3.*t4.*3.554762889834598e-13;
t92 = t4.*6.858999999999336e+3;
t94 = t4.*5.309999999993605e+2;
t95 = t4.*1.98899999999884e+3;
t97 = t4.*2.484000000001446e+3;
t98 = t4.*7.51000000000887e+2;
t7 = exp(t6);
t23 = t14.^2;
t24 = t15.^2;
t25 = t16.^2;
t27 = t8.^(3.77e+2./5.0e+2);
t28 = t21.^2;
t29 = t22.^2;
t30 = t8.^(3.11e+2./1.0e+3);
t31 = t8.^(8.77e+2./5.0e+2);
t32 = t8.^(4.89e+2./1.0e+3);
t33 = t8.^(9.93e+2./5.0e+2);
t34 = t8.^2.986;
t35 = t8.^4.646;
t36 = t8.^5.646;
t37 = 1.0./t8.^(2.09e+2./1.0e+3);
t38 = t8.^(7.91e+2./1.0e+3);
t39 = t8.^(8.03e+2./1.0e+3);
t40 = t8.^(9.89e+2./1.0e+3);
t41 = t8.^1.311;
t42 = t8.^1.409;
t43 = t8.^3.187;
t44 = t8.^6.844e-1;
t45 = t8.^4.187;
t46 = t8.^1.1444;
t47 = t8.^6.249;
t48 = t8.^7.249;
t49 = t8-7.164e-1;
t50 = t8-7.204e-1;
t51 = t8-1.5445;
t52 = t8-1.3444;
t54 = t8-1.4517;
t77 = t18-2.450088e-1;
t82 = t19-6.036356e-1;
t83 = t20-4.012628e-1;
t84 = t17-3.7860336e-1;
t90 = t26-1.2254063;
t96 = -t92;
t99 = -t94;
t100 = -t95;
t101 = -t97;
t102 = -t98;
t55 = t49.^2;
t56 = t50.^2;
t57 = t51.^2;
t58 = t52.^2;
t62 = t54.^2;
t63 = t23.*(4.89e+2./1.0e+3);
t64 = t25.*(1.03e+2./1.0e+3);
t66 = t28.*(3.37e+2./2.0e+2);
t67 = t24.*2.506;
t73 = t29.*1.607;
t78 = t40.*2.1101;
t91 = rho.*t46.*1.729249419654372e-4;
t103 = exp(t96);
t104 = exp(t99);
t105 = exp(t100);
t106 = exp(t101);
t107 = exp(t102);
t113 = t32.*4.52059;
t114 = t44.*6.93643;
t116 = rho.*t39.*9.447562548362136e-5;
t119 = t7.*t31.*7.77414e-1;
t126 = t2.*t42.*1.633921676808176e-9;
t129 = rho.*t7.*t31.*5.012986845499098e-5;
t131 = t2.*t7.*t41.*4.390189186720438e-9;
t132 = t3.*t7.*t41.*9.43639666993474e-14;
t65 = -t63;
t70 = -t64;
t71 = -t66;
t72 = -t67;
t74 = -t73;
t75 = t55.*(1.71e+2./1.0e+3);
t76 = t58.*2.245e-1;
t80 = t56.*2.785e-1;
t86 = t57.*3.967e-1;
t87 = t62.*1.304e-1;
t93 = -t91;
t108 = t103-1.0;
t109 = t104-1.0;
t110 = t105-1.0;
t111 = t106-1.0;
t112 = t107-1.0;
t115 = -t114;
t122 = -t119;
t133 = -t132;
t79 = -t75;
t81 = -t76;
t85 = -t80;
t88 = -t86;
t89 = -t87;
t117 = t65+t81;
t118 = t71+t79;
t121 = t72+t85;
t124 = t70+t89;
t128 = t74+t88;
t120 = exp(t117);
t123 = exp(t118);
t125 = exp(t121);
t127 = exp(t124);
t130 = exp(t128);
t134 = t36.*t120.*2.26312e-2;
t135 = t48.*t125.*2.31752e-2;
t137 = t34.*t130.*5.57346e-2;
t138 = rho.*t45.*t123.*2.730410110910498e-6;
t140 = t2.*t38.*t127.*4.015042715686892e-10;
t141 = rho.*t36.*t60.*t120.*1.459324219757545e-6;
t143 = rho.*t48.*t61.*t125.*1.494402888831571e-6;
t144 = rho.*t34.*t68.*t130.*3.593925715759608e-6;
t145 = t2.*t45.*t59.*t123.*8.803230948254119e-11;
t147 = t3.*t38.*t53.*t127.*8.630046246425269e-15;
t136 = -t135;
t139 = -t138;
t142 = -t141;
t146 = -t144;
t148 = -t147;
t149 = t69+t78+t93+t113+t115+t116+t122+t126+t129+t131+t133+t134+t136+t137+t139+t140+t142+t143+t145+t146+t148;
et1 = 1.0./t109.^2.*exp(t4.*(-1.061999999998721e+3)).*4.147575991701757e+2;
et2 = 1.0./t110.^2.*exp(t4.*(-3.977999999997681e+3)).*(-2.852060285124163e+3);
et3 = 1.0./t108.^2.*exp(t4.*(-1.371799999999867e+4)).*5.211660743085801e+4;
et4 = 1.0./t111.^2.*exp(t4.*(-4.968000000002893e+3)).*4.257320460091549e+3;
et5 = 1.0./t112.^2.*exp(t4.*(-1.502000000001774e+3)).*(-2.113609217775546e+2)+rho.*1.0./t8.^1.011.*1.480253927005417e-6;
et6 = rho.*1.0./t8.^1.511.*7.283985740327573e-5-rho.*1.0./t8.^1.3156.*9.661114093340211e-5-(t103.*5.211660743085801e+4)./t108;
et7 = (t104.*(-4.147575991701757e+2))./t109+(t105.*2.852060285124163e+3)./t110;
et8 = (t106.*(-4.257320460091549e+3))./t111+(t107.*2.113609217775546e+2)./t112;
et9 = t3.*1.0./t8.^(5.91e+2./1.0e+3).*(-2.023897381636773e-14)+t2.*1.0./t8.^1.197.*4.818543226360442e-10+t2.*1.0./t8.^8.556e-1.*9.213335645379665e-10;
et10 = 1.0./t4.^2.*1.365385267005982e-3+rho.*t7.*1.0./t8.^(1.23e+2./5.0e+2).*6.629755310962085e-5-rho.*t8.^(4.93e+2./5.0e+2).*t130.*2.131268390389476e-5;
et11 = rho.*t8.^3.646.*t120.*(-3.827999475491359e-5)+rho.*t8.^5.249.*t125.*6.769495795558421e-5;
et12 = t3.*t7.*1.0./t8.^(6.89e+2./1.0e+3).*(-3.847417086662462e-14)+t3.*1.0./t8.^1.209.*t127.*1.426710615412779e-15;
et13 = t2.*t8.^2.187.*t123.*1.174700408733436e-9+rho.*t36.*t120.*6.552365746711375e-7+rho.*t34.*t130.*2.851420662883673e-6;
et14 = rho.*t48.*t125.*(-8.323824090791849e-7)+t3.*t38.*t127.*2.25071606106771e-15-t2.*t45.*t123.*3.010704984302909e-11;
et15 = rho.*t35.*t82.*t120.*1.647868908950219e-5+rho.*t33.*t90.*t130.*2.146292437451638e-5-rho.*t47.*t83.*t125.*2.166585308228011e-5;
et16 = t2.*t43.*t77.*t123.*(-7.371825596068e-10)+t3.*t37.*t84.*t127.*1.365273316184478e-14-rho.*t36.*t82.^2.*t120.*1.459324219757545e-6;
et17 = rho.*t34.*t90.^2.*t130.*(-3.593925715759608e-6)+rho.*t48.*t83.^2.*t125.*1.494402888831571e-6+t2.*t45.*t77.^2.*t123.*8.803230948254119e-11-t3.*t38.*t84.^2.*t127.*8.630046246425269e-15;
et18 = t39.*1.465128-t46.*2.68172-t129+t132+rho.*t42.*5.067771472788238e-5+t2.*t4.*1.653817886866649e-8+t7.*t31.*1.554828-t45.*t123.*4.23432e-2+t53.*t147+t60.*t141+t68.*t144;
et19 = rho.*t7.*t41.*1.361661078153211e-4-rho.*t36.*t120.*1.427219086922879e-6-rho.*t34.*t130.*1.155087725045138e-5+rho.*t38.*t127.*1.245305648697446e-5;
et20 = rho.*t48.*t125.*7.489947278823833e-6-t2.*t7.*t41.*8.780378373440877e-9-t3.*t38.*t127.*1.777789526763605e-15;
et21 = t2.*t45.*t123.*2.966688829561638e-10-t36.*t60.*t120.*4.52624e-2-t34.*t68.*t130.*1.114692e-1+t48.*t61.*t125.*4.63504e-2;
et22 = rho.*t45.*t59.*t123.*5.460820221820995e-6-t2.*t38.*t53.*t127.*8.030085431373784e-10-rho.*t48.*t61.^2.*t125.*1.494402888831571e-6-t2.*t45.*t59.^2.*t123.*8.803230948254119e-11;
et23 = t3./9.32410994128e+13-t7.*t27.*1.363584156+t35.*t120.*1.277757552e-1+t33.*t130.*1.664235156e-1-t47.*t125.*1.679970248e-1+t77.*t138+t83.*t135;
et24 = t82.*t141+t84.*t147+t90.*t144+rho.*1.0./t8.^(1.97e+2./1.0e+3).*7.586392726334795e-5-rho.*t8.^1.444e-1.*1.978953035852463e-4+t2.*t8.^(4.09e+2./1.0e+3).*2.30219564262272e-9+1.0./t8.^(1.1e+1./1.0e+3).*2.0868889;
et25 = 1.0./t8.^(5.11e+2./1.0e+3).*2.21056851-1.0./t8.^3.156e-1.*4.747292692+rho.*t7.*t27.*8.792778927005417e-5-rho.*t43.*t123.*1.143222713438225e-5;
et26 = t2.*t7.*t30.*5.755538023790495e-9-t3.*t7.*t30.*1.237111603428444e-13+t2.*t37.*t127.*3.175898788108332e-10;
et27 = t36.*t82.*t120.*(-2.26312e-2)-t34.*t90.*t130.*5.57346e-2-rho.*t35.*t60.*t120.*8.239344544751096e-6-rho.*t33.*t68.*t130.*1.073146218725819e-5;
et28 = rho.*t47.*t61.*t125.*1.083292654114006e-5-t3.*t37.*t53.*t127.*6.826366580922388e-15+t2.*t43.*t59.*t123.*3.685912798034e-10;
et29 = t2.*t38.*t84.*t127.*(-4.015042715686892e-10)-rho.*t48.*t61.*t83.*t125.*1.494402888831571e-6-t2.*t45.*t59.*t77.*t123.*8.803230948254119e-11;
cp = ((t5.*t149-rho.*t4.*(et23+et24+et25+et26+et27+et28+et29).*2.137283982460665e-3+1.0).^2.*8.314472)./((t2.*(et18+et19+et20+et21+et22))./2.40498064e+8+(rho.*t149)./7.754e+3+1.0)+t4.^2.*(et1+et2+et3+et4+et5+et6+et7+et8+et9+et10+et11+et12+et13+et14+et15+et16+et17).*9.1342043168138e+3;

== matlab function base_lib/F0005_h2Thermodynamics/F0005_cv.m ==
function cv = F0005_cv(T,rho)
%ISOCHORICHEATCAPACITY
%    CV = ISOCHORICHEATCAPACITY(T,RHO)

%    This function was generated by the Symbolic Math Toolbox version 8.7.
%    04-Nov-2021 19:06:04

t2 = rho.^2;
t3 = rho.^3;
t4 = 1.0./T;
t5 = rho./1.5508e+4;
t6 = -t5;
t8 = t4.*3.3145e+1;
t9 = t5-3.9e+1./2.5e+2;
t10 = t5-6.7e+1./1.0e+2;
t11 = t5-2.17e+2./1.25e+2;
t12 = t4.*8.644216;
t13 = t4.*1.133559e+1;
t14 = t4.*1.4882105e+1;
t15 = t4.*1.8461765e+1;
t16 = t5-7.53e+2./5.0e+2;
t17 = t5-8.31e+2./5.0e+2;
t21 = t4.*2.6297243e+1;
t64 = t4.*6.858999999999336e+3;
t65 = t4.*5.309999999993605e+2;
t66 = t4.*1.98899999999884e+3;
t68 = t4.*2.484000000001446e+3;
t69 = t4.*7.51000000000887e+2;
t7 = exp(t6);
t18 = t9.^2;
t19 = t10.^2;
t20 = t11.^2;
t22 = t16.^2;
t23 = t17.^2;
t24 = t8.^2.986;
t25 = t8.^5.646;
t26 = t8.^(7.91e+2./1.0e+3);
t27 = t8.^4.187;
t28 = t8.^7.249;
t29 = t8-7.164e-1;
t30 = t8-7.204e-1;
t31 = t8-1.5445;
t32 = t8-1.3444;
t33 = t8-1.4517;
t51 = t13-2.450088e-1;
t55 = t14-6.036356e-1;
t56 = t15-4.012628e-1;
t57 = t12-3.7860336e-1;
t63 = t21-1.2254063;
t67 = -t64;
t70 = -t65;
t71 = -t66;
t72 = -t68;
t73 = -t69;
t34 = t29.^2;
t35 = t30.^2;
t36 = t31.^2;
t37 = t32.^2;
t38 = t33.^2;
t39 = t18.*(4.89e+2./1.0e+3);
t40 = t20.*(1.03e+2./1.0e+3);
t42 = t22.*(3.37e+2./2.0e+2);
t43 = t19.*2.506;
t47 = t23.*1.607;
t74 = exp(t67);
t75 = exp(t70);
t76 = exp(t71);
t77 = exp(t72);
t78 = exp(t73);
t41 = -t39;
t44 = -t40;
t45 = -t42;
t46 = -t43;
t48 = -t47;
t49 = t34.*(1.71e+2./1.0e+3);
t50 = t37.*2.245e-1;
t53 = t35.*2.785e-1;
t59 = t36.*3.967e-1;
t60 = t38.*1.304e-1;
t79 = t74-1.0;
t80 = t75-1.0;
t81 = t76-1.0;
t82 = t77-1.0;
t83 = t78-1.0;
t52 = -t49;
t54 = -t50;
t58 = -t53;
t61 = -t59;
t62 = -t60;
t84 = t41+t54;
t85 = t45+t52;
t87 = t46+t58;
t89 = t44+t62;
t92 = t48+t61;
t86 = exp(t84);
t88 = exp(t85);
t90 = exp(t87);
t91 = exp(t89);
t93 = exp(t92);
et1 = 1.0./t80.^2.*exp(t4.*(-1.061999999998721e+3)).*4.147575991701757e+2;
et2 = 1.0./t81.^2.*exp(t4.*(-3.977999999997681e+3)).*(-2.852060285124163e+3);
et3 = 1.0./t79.^2.*exp(t4.*(-1.371799999999867e+4)).*5.211660743085801e+4;
et4 = 1.0./t82.^2.*exp(t4.*(-4.968000000002893e+3)).*4.257320460091549e+3;
et5 = 1.0./t83.^2.*exp(t4.*(-1.502000000001774e+3)).*(-2.113609217775546e+2)+rho.*1.0./t8.^1.011.*1.480253927005417e-6;
et6 = rho.*1.0./t8.^1.511.*7.283985740327573e-5-rho.*1.0./t8.^1.3156.*9.661114093340211e-5-(t74.*5.211660743085801e+4)./t79;
et7 = (t75.*(-4.147575991701757e+2))./t80+(t76.*2.852060285124163e+3)./t81;
et8 = (t77.*(-4.257320460091549e+3))./t82+(t78.*2.113609217775546e+2)./t83;
et9 = t3.*1.0./t8.^(5.91e+2./1.0e+3).*(-2.023897381636773e-14)+t2.*1.0./t8.^1.197.*4.818543226360442e-10+t2.*1.0./t8.^8.556e-1.*9.213335645379665e-10;
et10 = 1.0./t4.^2.*1.365385267005982e-3+rho.*t7.*1.0./t8.^(1.23e+2./5.0e+2).*6.629755310962085e-5-rho.*t8.^(4.93e+2./5.0e+2).*t93.*2.131268390389476e-5;
et11 = rho.*t8.^3.646.*t86.*(-3.827999475491359e-5)+rho.*t8.^5.249.*t90.*6.769495795558421e-5;
et12 = t3.*t7.*1.0./t8.^(6.89e+2./1.0e+3).*(-3.847417086662462e-14)+t3.*1.0./t8.^1.209.*t91.*1.426710615412779e-15;
et13 = t2.*t8.^2.187.*t88.*1.174700408733436e-9+rho.*t25.*t86.*6.552365746711375e-7+rho.*t24.*t93.*2.851420662883673e-6;
et14 = rho.*t28.*t90.*(-8.323824090791849e-7)-t2.*t27.*t88.*3.010704984302909e-11+t3.*t26.*t91.*2.25071606106771e-15;
et15 = rho.*t25.*t55.^2.*t86.*(-1.459324219757545e-6)+rho.*t28.*t56.^2.*t90.*1.494402888831571e-6-rho.*t24.*t63.^2.*t93.*3.593925715759608e-6+rho.*t8.^(9.93e+2./5.0e+2).*t63.*t93.*2.146292437451638e-5;
et16 = rho.*t8.^4.646.*t55.*t86.*1.647868908950219e-5-rho.*t8.^6.249.*t56.*t90.*2.166585308228011e-5+t2.*t27.*t51.^2.*t88.*8.803230948254119e-11;
et17 = t3.*t26.*t57.^2.*t91.*(-8.630046246425269e-15)+t3.*1.0./t8.^(2.09e+2./1.0e+3).*t57.*t91.*1.365273316184478e-14-t2.*t8.^3.187.*t51.*t88.*7.371825596068e-10;
cv = t4.^2.*(et1+et2+et3+et4+et5+et6+et7+et8+et9+et10+et11+et12+et13+et14+et15+et16+et17).*9.1342043168138e+3;

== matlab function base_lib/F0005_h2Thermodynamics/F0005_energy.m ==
function u = F0005_energy(T,rho)
%INTERNALENERGY
%    U = INTERNALENERGY(T,RHO)

%    This function was generated by the Symbolic Math Toolbox version 8.7.
%    04-Nov-2021 19:06:03

t2 = rho.^2;
t3 = rho.^3;
t4 = 1.0./T;
t5 = rho./1.5508e+4;
t6 = -t5;
t8 = t4.*3.3145e+1;
t9 = t5-3.9e+1./2.5e+2;
t10 = t5-6.7e+1./1.0e+2;
t11 = t5-2.17e+2./1.25e+2;
t12 = t5-7.53e+2./5.0e+2;
t13 = t5-8.31e+2./5.0e+2;
t49 = t4.*6.858999999999336e+3;
t50 = t4.*5.309999999993605e+2;
t51 = t4.*1.98899999999884e+3;
t53 = t4.*2.484000000001446e+3;
t54 = t4.*7.51000000000887e+2;
t7 = exp(t6);
t14 = t9.^2;
t15 = t10.^2;
t16 = t11.^2;
t17 = t12.^2;
t18 = t13.^2;
t19 = t8-7.164e-1;
t20 = t8-7.204e-1;
t21 = t8-1.5445;
t22 = t8-1.3444;
t23 = t8-1.4517;
t52 = -t49;
t55 = -t50;
t56 = -t51;
t57 = -t53;
t58 = -t54;
t24 = t19.^2;
t25 = t20.^2;
t26 = t21.^2;
t27 = t22.^2;
t28 = t23.^2;
t29 = t14.*(4.89e+2./1.0e+3);
t30 = t16.*(1.03e+2./1.0e+3);
t32 = t17.*(3.37e+2./2.0e+2);
t33 = t15.*2.506;
t37 = t18.*1.607;
t59 = exp(t52);
t60 = exp(t55);
t61 = exp(t56);
t62 = exp(t57);
t63 = exp(t58);
t31 = -t29;
t34 = -t30;
t35 = -t32;
t36 = -t33;
t38 = -t37;
t39 = t24.*(1.71e+2./1.0e+3);
t40 = t27.*2.245e-1;
t42 = t25.*2.785e-1;
t45 = t26.*3.967e-1;
t46 = t28.*1.304e-1;
t41 = -t39;
t43 = -t40;
t44 = -t42;
t47 = -t45;
t48 = -t46;
t64 = t31+t43;
t65 = t35+t41;
t67 = t36+t44;
t69 = t34+t48;
t72 = t38+t47;
t66 = exp(t64);
t68 = exp(t65);
t70 = exp(t67);
t71 = exp(t69);
t73 = exp(t72);
et1 = T.*1.2471708e+1-(t59.*6.940424851620928e+4)./(t59-1.0);
et2 = (t60.*(-7.134615165303407e+3))./(t60-1.0)+(t61.*1.309768796792836e+4)./(t61-1.0);
et3 = (t62.*(-1.565508652359312e+4))./(t62-1.0)+(t63.*2.570724159925436e+3)./(t63-1.0);
et4 = rho.*1.0./t8.^(1.1e+1./1.0e+3).*3.708482510740261e-2+rho.*1.0./t8.^(5.11e+2./1.0e+3).*3.928265974354533e-2;
et5 = rho.*1.0./t8.^3.156e-1.*(-8.436123227090361e-2)+t2.*1.0./t8.^(1.97e+2./1.0e+3).*6.740657048206955e-7;
et6 = t3.*t8.^(4.09e+2./1.0e+3).*1.363696980861286e-11-t2.*t8.^1.444e-1.*1.758338147046353e-6;
et7 = t2.^2.*4.764633820313524e-17-rho.*t7.*t8.^(3.77e+2./5.0e+2).*2.42314192885329e-2;
et8 = rho.*t8.^(9.93e+2./5.0e+2).*t73.*2.957410415947438e-3+rho.*t8.^4.646.*t66.*2.270624724947404e-3;
et9 = rho.*t8.^6.249.*t70.*(-2.985372284682706e-3)+t3.*1.0./t8.^(2.09e+2./1.0e+3).*t71.*1.881231772261721e-12;
et10 = t3.*t7.*t8.^(3.11e+2./1.0e+3).*3.409271428093691e-11;
et11 = t2.*t8.^3.187.*t68.*(-1.015775549591232e-7);
et12 = rho.*t8.^5.646.*t66.*(t4.*1.4882105e+1-6.036356e-1).*(-4.021652010179603e-4);
et13 = rho.*t8.^7.249.*t70.*(t4.*1.8461765e+1-4.012628e-1).*4.118322919965107e-4;
et14 = t2.*t8.^4.187.*t68.*(t4.*1.133559e+1-2.450088e-1).*2.426022330048322e-8;
et15 = t3.*t8.^(7.91e+2./1.0e+3).*t71.*(t4.*8.644216-3.7860336e-1).*(-2.378295540153882e-12);
et16 = rho.*t8.^2.986.*t73.*(t4.*2.6297243e+1-1.2254063).*(-9.90425457450582e-4)+5.203221931700199e+2;
u = et1+et2+et3+et4+et5+et6+et7+et8+et9+et10+et11+et12+et13+et14+et15+et16;

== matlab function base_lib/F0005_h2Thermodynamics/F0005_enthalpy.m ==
function h = F0005_enthalpy(T,rho)
%ENTHALPY
%    H = ENTHALPY(T,RHO)

%    This function was generated by the Symbolic Math Toolbox version 8.7.
%    04-Nov-2021 19:06:04

t2 = rho.^2;
t3 = rho.^3;
t4 = 1.0./T;
t5 = rho./1.5508e+4;
t6 = -t5;
t8 = t4.*3.3145e+1;
t9 = t5-3.9e+1./2.5e+2;
t10 = t5-6.7e+1./1.0e+2;
t11 = t5-2.17e+2./1.25e+2;
t12 = t5-7.53e+2./5.0e+2;
t13 = t5-8.31e+2./5.0e+2;
t56 = t4.*6.858999999999336e+3;
t57 = t4.*5.309999999993605e+2;
t58 = t4.*1.98899999999884e+3;
t60 = t4.*2.484000000001446e+3;
t61 = t4.*7.51000000000887e+2;
t7 = exp(t6);
t14 = t9.^2;
t15 = t10.^2;
t16 = t11.^2;
t17 = t12.^2;
t18 = t13.^2;
t19 = t8.^(8.77e+2./5.0e+2);
t20 = t8.^2.986;
t21 = t8.^5.646;
t22 = t8.^(7.91e+2./1.0e+3);
t23 = t8.^1.311;
t24 = t8.^4.187;
t25 = t8.^7.249;
t26 = t8-7.164e-1;
t27 = t8-7.204e-1;
t28 = t8-1.5445;
t29 = t8-1.3444;
t30 = t8-1.4517;
t59 = -t56;
t62 = -t57;
t63 = -t58;
t64 = -t60;
t65 = -t61;
t31 = t26.^2;
t32 = t27.^2;
t33 = t28.^2;
t34 = t29.^2;
t35 = t30.^2;
t36 = t14.*(4.89e+2./1.0e+3);
t37 = t16.*(1.03e+2./1.0e+3);
t39 = t17.*(3.37e+2./2.0e+2);
t40 = t15.*2.506;
t44 = t18.*1.607;
t66 = exp(t59);
t67 = exp(t62);
t68 = exp(t63);
t69 = exp(t64);
t70 = exp(t65);
t38 = -t36;
t41 = -t37;
t42 = -t39;
t43 = -t40;
t45 = -t44;
t46 = t31.*(1.71e+2./1.0e+3);
t47 = t34.*2.245e-1;
t49 = t32.*2.785e-1;
t52 = t33.*3.967e-1;
t53 = t35.*1.304e-1;
t48 = -t46;
t50 = -t47;
t51 = -t49;
t54 = -t52;
t55 = -t53;
t71 = t38+t50;
t72 = t42+t48;
t74 = t43+t51;
t76 = t41+t55;
t79 = t45+t54;
t73 = exp(t71);
t75 = exp(t72);
t77 = exp(t74);
t78 = exp(t76);
t80 = exp(t79);
et1 = T.*4.525569467491326e-2-(t66.*2.518450143309456e+2)./(t66-1.0)-(t67.*2.58891537184784e+1)./(t67-1.0)+(t68.*4.75271685020088e+1)./(t68-1.0)-(t69.*5.68071202293286e+1)./(t69-1.0);
et2 = (t70.*9.32830592850702)./(t70-1.0)+rho.*1.0./t8.^(1.1e+1./1.0e+3).*1.345685388186742e-4+rho.*1.0./t8.^(5.11e+2./1.0e+3).*1.425437522568997e-4-rho.*1.0./t8.^3.156e-1.*3.061189509930358e-4;
et3 = t2.*1.0./t8.^(1.97e+2./1.0e+3).*2.445961028609361e-9+t3.*t8.^(4.09e+2./1.0e+3).*4.94840435608013e-14-t2.*t8.^1.444e-1.*6.380426347215835e-9+t2.^2./5.78393187877481e+18;
et4 = rho.*t7.*t8.^(3.77e+2./5.0e+2).*(-8.792778927005417e-5)+rho.*t8.^(9.93e+2./5.0e+2).*t80.*1.073146218725819e-5+rho.*t8.^4.646.*t73.*8.239344544751096e-6;
et5 = rho.*t8.^6.249.*t77.*(-1.083292654114006e-5)+t3.*1.0./t8.^(2.09e+2./1.0e+3).*t78.*6.826366580922388e-15+t3.*t7.*t8.^(3.11e+2./1.0e+3).*1.237111603428444e-13;
et6 = t2.*t8.^3.187.*t75.*(-3.685912798034e-10)-rho.*t21.*t73.*(t4.*1.4882105e+1-6.036356e-1).*1.459324219757545e-6;
et7 = rho.*t25.*t77.*(t4.*1.8461765e+1-4.012628e-1).*1.494402888831571e-6+t2.*t24.*t75.*(t4.*1.133559e+1-2.450088e-1).*8.803230948254119e-11;
et8 = t3.*t22.*t78.*(t4.*8.644216-3.7860336e-1).*(-8.630046246425269e-15)-rho.*t20.*t80.*(t4.*2.6297243e+1-1.2254063).*3.593925715759608e-6+1.888076782;
et9 = t3.*t4.*3.554762889834598e-13-t7.*t19.*7.77414e-1+t21.*t73.*2.26312e-2+t20.*t80.*5.57346e-2-t25.*t77.*2.31752e-2;
et10 = rho.*t8.^(8.03e+2./1.0e+3).*9.447562548362136e-5-rho.*t8.^1.1444.*1.729249419654372e-4+t2.*t8.^1.409.*1.633921676808176e-9+t8.^(4.89e+2./1.0e+3).*4.52059;
et11 = t8.^(9.89e+2./1.0e+3).*2.1101-t8.^6.844e-1.*6.93643+rho.*t7.*t19.*5.012986845499098e-5-rho.*t24.*t75.*2.730410110910498e-6+t2.*t7.*t23.*4.390189186720438e-9;
et12 = t3.*t7.*t23.*(-9.43639666993474e-14)+t2.*t22.*t78.*4.015042715686892e-10+rho.*t25.*t77.*(rho.*3.231880319834924e-4-3.35804).*1.494402888831571e-6;
et13 = rho.*t21.*t73.*(rho.*6.30642249161723e-5-1.52568e-1).*(-1.459324219757545e-6)-rho.*t20.*t80.*(rho.*2.072478720660304e-4-5.341668).*3.593925715759608e-6;
et14 = t2.*t24.*t75.*(rho.*2.17307196285788e-4-5.07522).*8.803230948254119e-11-t3.*t22.*t78.*(rho.*1.328346659788496e-5-3.57616e-1).*8.630046246425269e-15;
h = T.*(t8.*(et1+et2+et3+et4+et5+et6+et7+et8)+t5.*(et9+et10+et11+et12+et13+et14)+1.0).*8.314472;
